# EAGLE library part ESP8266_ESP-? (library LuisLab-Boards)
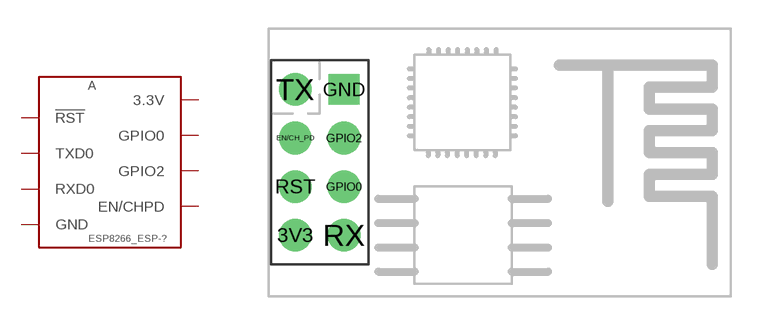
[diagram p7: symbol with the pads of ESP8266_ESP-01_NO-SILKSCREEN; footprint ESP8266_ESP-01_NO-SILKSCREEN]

Designator prefix A

## ESP8266_ESP-01  [ESP8266_ESP-01_NO-SILKSCREEN]
3V3  3.3V  pas
EN/CH_PD  EN/CHPD
GND  GND  pas
GPIO0  GPIO0
GPIO2  GPIO2
RST  !RST!
RX  RXD0
TX  TXD0

## Footprint ESP8266_ESP-01_NO-SILKSCREEN (pad centres in mm)
ESP8266 ESP-01, No-Silkscreen delimiting the board
drill 1.016 pad 1.7: 3V3 -1.27,-3.81; EN/CH_PD -1.27,1.27; GPIO0 1.27,-1.27; GPIO2 1.27,1.27; RST -1.27,-1.27; RX 1.27,-3.81; TX -1.27,3.81
drill 1.016 pad 1.6 square: GND 1.27,3.81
